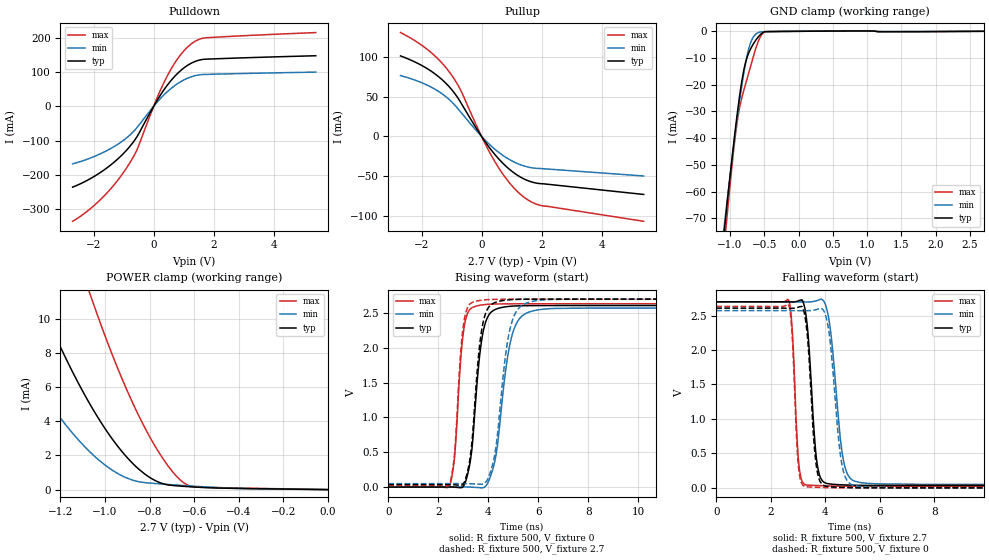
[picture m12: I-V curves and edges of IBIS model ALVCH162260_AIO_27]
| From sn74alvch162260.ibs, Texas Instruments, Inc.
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[Model]   ALVCH162260_AIO_27
Model_type  I/O
Vinl=0.8
Vinh=2.0
Enable   Active-Low
Vref =   0
Rref =   500
Cref =   50p
Vmeas =   1.5
| variable   typ   min   max
C_comp   8.54pF   7.35pF   9.56pF
| C_pullup   9.71pF   8.11pF   10.67pF
| C_pulldown   13.00pF   10.17pF   16.97pF
| C_tri-state   8.54pF   7.35pF   9.56pF
[Temperature Range]   40   100   -40
| Ambient temperature   25   85   -40
[Voltage range]   2.7   2.7   2.7
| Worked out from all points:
|   slope of the pulldown table from 0 to 0.405 V, typ, clamps not added: 7.25 ohm
|   slope of the pullup table from 0 to 0.405 V, typ, clamps not added: 19.2 ohm
|   GND clamp passes 1 mA (typ) near -0.55 V on its own axis
|   POWER clamp passes 1 mA (typ) near -0.83 V on its own axis
|   rising waveform, R_fixture 500, V_fixture 0: 20-80 % time 389ps typ, 537ps min, 292ps max; typ from 0 V to 2.61 V
|   falling waveform, R_fixture 500, V_fixture 2.7: 20-80 % time 259ps typ, 370ps min, 182ps max; typ from 2.7 V to 0.034 V
|   rising waveform, R_fixture 500, V_fixture 2.7: 20-80 % time 376ps typ, 504ps min, 284ps max; typ from 0.034 V to 2.7 V
|   falling waveform, R_fixture 500, V_fixture 0: 20-80 % time 247ps typ, 346ps min, 173ps max; typ from 2.61 V to 0 V
[GND Clamp]
| ALVCH162260_AIO_27
|   Voltage   I(typ)   I(min)   I(max)
-2.7V     -526.4mA   -481.2mA   -596.1mA
-1.095V   -77.41mA   -75.39mA   -83.81mA
-1.075V   -72.44mA   -70.89mA   -78.17mA
-1.055V   -67.52mA   -66.42mA   -72.6mA
-915mV    -35.16mA   -36.7mA    -37.62mA
-870mV    -26.08mA   -27.99mA   -29.9mA
-810mV    -16.08mA   -17.49mA   -23.16mA
-765mV    -10.95mA   -10.89mA   -18.99mA
-705mV    -6.866mA   -4.674mA   -13.59mA
-595mV    -2.326mA   -581.8uA   -4.241mA
-480mV    -124.9uA   -135.1uA   -159.8uA
2.7V      95.48pA    346.5pA    50.89pA
[POWER Clamp]
| ALVCH162260_AIO_27
|   Voltage   I(typ)   I(min)   I(max)
-2.7V     73.72mA    50.39mA    108.2mA
-1.525V   19mA       11.2mA     32.77mA
-1.31V    11.61mA    6.263mA    21.89mA
-1.29V    10.99mA    5.862mA    20.95mA
-1.17V    7.535mA    3.692mA    15.6mA
-1.065V   4.947mA    2.175mA    11.38mA
-945mV    2.572mA    959.4uA    7.168mA
-845mV    1.159mA    451.1uA    4.233mA
-750mV    387.8uA    333.2uA    2.01mA
-655mV    199.1uA    246.5uA    483.8uA
-600mV    151.5uA    199.7uA    159.3uA
-35.59fV  95.48pA    346.5pA    50.89pA
[Pulldown]
| ALVCH162260_AIO_27
|   Voltage   I(typ)   I(min)   I(max)
-2.7V     -236.1mA   -167.9mA   -335.8mA
-2.22V    -216.5mA   -154.7mA   -306.9mA
-1.755V   -192mA     -137.8mA   -271mA
-1.32V    -163.3mA   -117.6mA   -229.4mA
-930mV    -130.8mA   -94.13mA   -183.5mA
-555mV    -88.6mA    -61.97mA   -126.8mA
80mV      12.19mA    8.473mA    17.55mA
450mV     61.21mA    42.38mA    88.22mA
845mV     100.2mA    69.06mA    144.7mA
1.245V    125.7mA    86.07mA    182mA
1.725V    137.7mA    93.27mA    200.2mA
5.4V      147.8mA    100mA      215.5mA
[Pullup]
| ALVCH162260_AIO_27
|   Voltage   I(typ)   I(min)   I(max)
-2.7V     101.7mA    76.83mA    131.2mA
-1.775V   84.75mA    64.08mA    108.9mA
-1.4V     74.43mA    56mA       95.88mA
-1.075V   62.56mA    46.48mA    81.41mA
-695mV    42.89mA    30.71mA    58.34mA
25mV      -1.44mA    -1.029mA   -1.994mA
445mV     -22.91mA   -16.26mA   -31.97mA
920mV     -41.28mA   -29.03mA   -58.17mA
1.395V    -53.38mA   -37.07mA   -76.22mA
1.695V    -57.79mA   -39.72mA   -83.43mA
2V        -59.73mA   -40.65mA   -87.44mA
5.4V      -73.3mA    -49.98mA   -107.2mA
[Ramp]
| ALVCH162260_AIO_27
| variable   typ   min   max
dV/dt_r   1.57/3.95E-10   1.55/5.44E-10   1.59/3.05E-10
dV/dt_f   1.62/2.68E-10   1.61/3.85E-10   1.63/1.90E-10
R_load = 500
[Rising Waveform]
| ALVCH162260_AIO_27
R_fixture =   500
C_fixture =   0
L_fixture =   0
V_fixture =   0
V_fixture_min = 0
V_fixture_max = 0
|   Time   V(typ)   V(min)   V(max)
0s        369pV      1.332nV    255.5pV
2.45ns    1.685mV    -92.63uV   18.23mV
2.65ns    -1.712mV   573.4uV    429.4mV
3.02ns    19.41mV    1.384mV    2.263V
3.345ns   542.4mV    -1.88mV    2.576V
3.75ns    2.141V     -11.52mV   2.617V
4.27ns    2.55V      384.6mV    2.63V
4.995ns   2.6V       2.231V     2.633V
6.005ns   2.607V     2.547V     2.633V
50ns      2.608V     2.572V     2.633V
[Falling Waveform]
| ALVCH162260_AIO_27
R_fixture =   500
C_fixture =   0
L_fixture =   0
V_fixture =   2.7
V_fixture_min = 2.7
V_fixture_max = 2.7
|   Time   V(typ)   V(min)   V(max)
0s        2.7V       2.7V       2.7V
2.67ns    2.698V     2.7V       2.714V
3.03ns    2.716V     2.698V     347.5mV
3.34ns    2.355V     2.697V     39.43mV
3.635ns   594.2mV    2.71V      35.11mV
3.8ns     172.2mV    2.732V     32.2mV
4.155ns   57.5mV     2.398V     27.16mV
4.695ns   42.82mV    348.2mV    24.76mV
5.31ns    36.66mV    75.18mV    24.2mV
50ns      34.45mV    49.51mV    23.96mV
[Rising Waveform]
| ALVCH162260_AIO_27
R_fixture =   500
C_fixture =   0
L_fixture =   0
V_fixture =   2.7
V_fixture_min = 2.7
V_fixture_max = 2.7
|   Time   V(typ)   V(min)   V(max)
0s        34.45mV    49.51mV    23.96mV
2.45ns    35.67mV    49.51mV    43.65mV
2.645ns   32.06mV    50.08mV    455mV
3.04ns    69.62mV    50.07mV    2.404V
3.32ns    556.5mV    46.93mV    2.644V
3.705ns   2.182V     39.84mV    2.683V
4.245ns   2.647V     433.9mV    2.696V
4.935ns   2.692V     2.359V     2.699V
5.895ns   2.699V     2.676V     2.7V
50ns      2.7V       2.7V       2.7V
[Falling Waveform]
| ALVCH162260_AIO_27
R_fixture =   500
C_fixture =   0
L_fixture =   0
V_fixture =   0
V_fixture_min = 0
V_fixture_max = 0
|   Time   V(typ)   V(min)   V(max)
0s        2.608V     2.572V     2.633V
2.665ns   2.606V     2.572V     2.648V
2.79ns    2.606V     2.571V     2.189V
3.01ns    2.622V     2.57V      337.3mV
3.295ns   2.384V     2.57V      15.12mV
3.775ns   128.8mV    2.599V     7.471mV
4.145ns   18.29mV    2.241V     2.682mV
4.63ns    7.516mV    304mV      736.4uV
5.205ns   2.141mV    22.64mV    232.5uV
50ns      215.9nV    356.6nV    115nV
